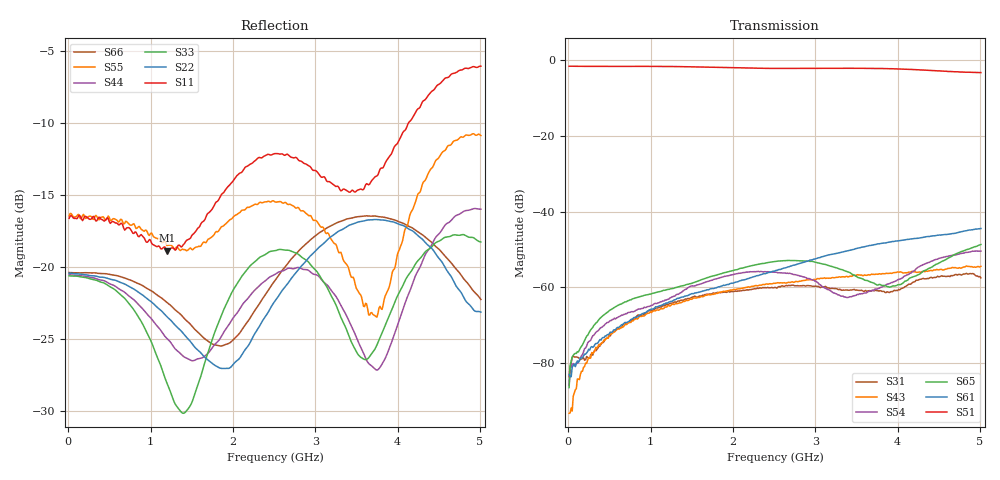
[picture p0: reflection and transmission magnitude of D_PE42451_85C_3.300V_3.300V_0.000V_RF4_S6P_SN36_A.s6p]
! Device ID: PE42451
! Serial: 36
! Insertion: A
! Temp: 85C
! VDD: 3.300
! Control_Hi: 100.000
! Control_Lo: 0.000
! Logic State: RF4
! Port 1: RFC
! Port 2: RF1
! Port 3: RF2
! Port 4: RF3
! Port 5: RF4
! Port 6: RF5
! V1 = 0.00
! V2 = 0.00
! V3 = 3.30
! V4 = 0.00
! IDD: 1.690750e-05
#  Hz  S  RI  R  50
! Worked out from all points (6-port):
!   401 points, 10 MHz to 5.01 GHz, reference 50 ohm
!   strongest paths, dB at 10 MHz, 1.26 GHz, 2.51 GHz, 3.76 GHz, 5.01 GHz:
!     S51: -1.6, -1.7, -2.2, -2.2, -3.3
!     S61: -83.1, -63.8, -55.7, -48.5, -44.5
!     S65: -86.5, -60.4, -53.2, -59.4, -48.7
!     S54: -85.9, -62.6, -56.1, -60.4, -50.5
!     S43: -93.3, -64.5, -59.0, -56.6, -54.5
!     S31: -83.6, -64.2, -60.0, -60.9, -57.5
!   lowest |S11| = -18.9 dB at 1.198 GHz (marker M1), VSWR 1.26, Z = 56 - j10.6 ohm
!   |S11| at or under -10 dB: start of sweep to 4.13 GHz
